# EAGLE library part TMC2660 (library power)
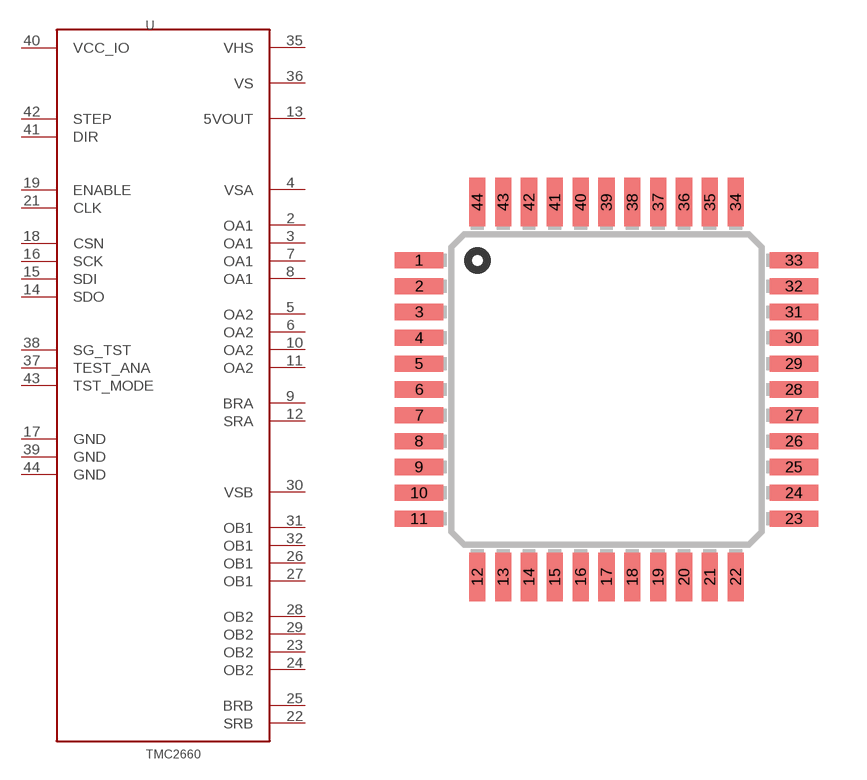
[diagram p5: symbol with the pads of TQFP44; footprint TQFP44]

Designator prefix U

## TMC2660U  [TQFP44]
2  OA1
3  OA1
4  VSA
5  OA2
6  OA2
7  OA1
8  OA1
9  BRA
10  OA2
11  OA2
12  SRA
13  5VOUT
14  SDO
15  SDI
16  SCK
17  GND
18  CSN
19  ENABLE
21  CLK
22  SRB
23  OB2
24  OB2
25  BRB
26  OB1
27  OB1
28  OB2
29  OB2
30  VSB
31  OB1
32  OB1
35  VHS
36  VS
37  TEST_ANA
38  SG_TST
39  GND
40  VCC_IO
41  DIR
42  STEP
43  TST_MODE
44  GND

## Footprint TQFP44 (pad centres in mm)
44-lead Thin Quad Flat Package
smd 1.5 x 0.5: 1 -5.8,4; 2 -5.8,3.2; 3 -5.8,2.4; 4 -5.8,1.6; 5 -5.8,0.8; 6 -5.8,0; 7 -5.8,-0.8; 8 -5.8,-1.6; 9 -5.8,-2.4; 10 -5.8,-3.2; 11 -5.8,-4; 23 5.8,-4; 24 5.8,-3.2; 25 5.8,-2.4; 26 5.8,-1.6; 27 5.8,-0.8; 28 5.8,0; 29 5.8,0.8; 30 5.8,1.6; 31 5.8,2.4; 32 5.8,3.2; 33 5.8,4
smd 0.5 x 1.5: 12 -4,-5.8; 13 -3.2,-5.8; 14 -2.4,-5.8; 15 -1.6,-5.8; 16 -0.8,-5.8; 17 0,-5.8; 18 0.8,-5.8; 19 1.6,-5.8; 20 2.4,-5.8; 21 3.2,-5.8; 22 4,-5.8; 34 4,5.8; 35 3.2,5.8; 36 2.4,5.8; 37 1.6,5.8; 38 0.8,5.8; 39 0,5.8; 40 -0.8,5.8; 41 -1.6,5.8; 42 -2.4,5.8; 43 -3.2,5.8; 44 -4,5.8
